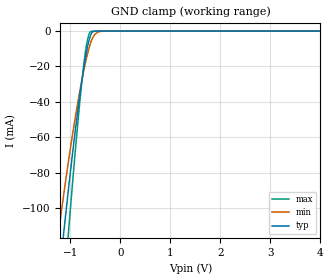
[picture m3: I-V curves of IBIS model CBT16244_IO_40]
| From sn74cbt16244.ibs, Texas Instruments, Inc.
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[Model]   CBT16244_IO_40
Model_type  Terminator
| variable   typ   min   max
C_comp   3.35pF   2.76pF   4.15pF
| C_tri-state   3.35pF   2.76pF   4.15pF
[Temperature Range]   40   100   -40
| Ambient temperature   25   85   -40
[Voltage range]   4   4   4
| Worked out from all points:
|   GND clamp passes 1 mA (typ) near -0.57 V on its own axis
[GND Clamp]
| CBT16244_IO_40
|   Voltage   I(typ)   I(min)   I(max)
-4V       -3.006A    -3.083A    -2.663A
-1.245V   -144.4mA   -115.7mA   -188.8mA
-1.18V    -126.4mA   -101.7mA   -164.4mA
-1.105V   -106.2mA   -86.31mA   -137mA
-1.03V    -86.88mA   -71.71mA   -110.4mA
-840mV    -42.12mA   -38.26mA   -48.02mA
-735mV    -21.16mA   -22.53mA   -19.25mA
-655mV    -8.489mA   -12.47mA   -4.434mA
-580mV    -1.347mA   -5.382mA   -55.45uA
-505mV    -73.79uA   -1.647mA   -2.79uA
-370mV    -991.9nA   -60.29uA   -12.88nA
4V        53.99pA    3.024nA    23.81pA
